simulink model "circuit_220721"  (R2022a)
settings: Solver=VariableStepAuto  StartTime=-D+0.1e-6  StopTime=34e-6  FixedStep=1e-3  MaxStep=0.1e-6  RelTol=1e-3
model workspace (MATLAB code in the model file):
  sGeo = CreateGeometry()
  sConst = CreateConstants()
libraries: fl_lib x9, nesl_utility x3, ee_lib x1

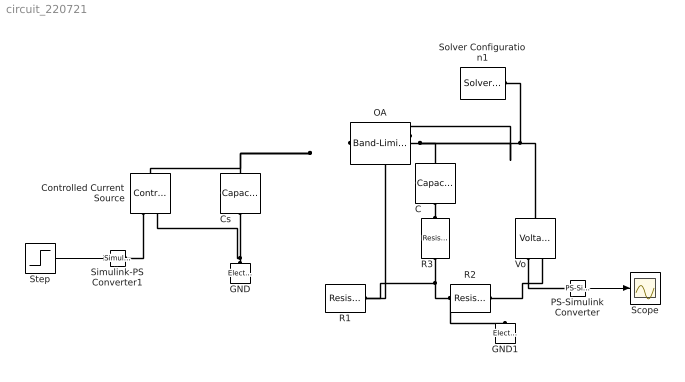
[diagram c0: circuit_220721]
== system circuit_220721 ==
  C : fl_lib/Electrical/Electrical Elements/Capacitor  c=100 uF  r=1e-6 Ohm  g=0 1/Ohm  i_specify=off  i_priority=None  i=0 A  i_nominal_specify=off  i_nominal_unit=A  i_nominal_value=1  v_specify=off  v_priority=None  v=0 V  v_nominal_specify=off  v_nominal_unit=V  v_nominal_value=1  vc_specify=off  vc_priority=High  vc=0 V  vc_nominal_specify=off  vc_nominal_unit=V  vc_nominal_value=1
  Controlled Current Source : fl_lib/Electrical/Electrical Sources/Controlled Current Source
  Cs : fl_lib/Electrical/Electrical Elements/Capacitor  c=33 pF  r=1e-6 Ohm  g=0 1/Ohm  i_specify=off  i_priority=None  i=0 A  i_nominal_specify=off  i_nominal_unit=A  i_nominal_value=1  v_specify=off  v_priority=None  v=0 V  v_nominal_specify=off  v_nominal_unit=V  v_nominal_value=1  vc_specify=off  vc_priority=High  vc=0 V  vc_nominal_specify=off  vc_nominal_unit=V  vc_nominal_value=1
  GND : fl_lib/Electrical/Electrical Elements/Electrical Reference
  GND1 : fl_lib/Electrical/Electrical Elements/Electrical Reference
  OA : ee_lib/Integrated Circuits/Band-Limited Op-Amp  A=100000  Rin=1e8 Ohm  Rout=0 Ohm  Vmin=-15 V  Vmax=15 V  Vdotmax=1000000 V/s  f=1 Hz  V0=0 V
  PS-Simulink Converter : nesl_utility/PS-Simulink Converter  PhysicalDomain=network_engine_domain  SubClassName=ps_output  LeftPortType=input  RightPortType=output  PseudoPeriodic=off  Frequencies=[]  VectorFormat=1-D array  Unit=inherit  AffineConversion=off
  R1 : fl_lib/Electrical/Electrical Elements/Resistor  R=10 MOhm  i_specify=off  i_priority=None  i=0 A  i_nominal_specify=off  i_nominal_unit=A  i_nominal_value=1  v_specify=off  v_priority=None  v=0 V  v_nominal_specify=off  v_nominal_unit=V  v_nominal_value=1
  R2 : fl_lib/Electrical/Electrical Elements/Resistor  R=100 kOhm  i_specify=off  i_priority=None  i=0 A  i_nominal_specify=off  i_nominal_unit=A  i_nominal_value=1  v_specify=off  v_priority=None  v=0 V  v_nominal_specify=off  v_nominal_unit=V  v_nominal_value=1
  R3 : fl_lib/Electrical/Electrical Elements/Resistor  R=1 kOhm  i_specify=off  i_priority=None  i=0 A  i_nominal_specify=off  i_nominal_unit=A  i_nominal_value=1  v_specify=off  v_priority=None  v=0 V  v_nominal_specify=off  v_nominal_unit=V  v_nominal_value=1
  Scope : Scope
  Simulink-PS Converter1 : nesl_utility/Simulink-PS Converter  PhysicalDomain=network_engine_domain  SubClassName=ps_input  LeftPortType=input  RightPortType=output  PseudoPeriodic=off  Frequencies=[]  NoiseDistribution=none  NoiseParameters=[]  Unit=1  AffineConversion=off  FilteringAndDerivatives=provide  SimscapeFilterOrder=1  InputFilterTimeConstant=0.001  UdotUserProvided=0
  Solver Configuration1 : nesl_utility/Solver Configuration  PhysicalDomain=network_engine_domain  SubClassName=solver  LeftPortType=input  RightPortType=generic  Tones=[]  Harmonics=[]  SimulateNoise=off  Profile=off  UseLocalSampling=off  EnableSwitchedLinearOptims=on  FrequencyDomain=off  UseCCode=off  RelTol=0.001  AbsTol=1e-06  MinStep=1e-09  ToWorkspace=off  RevertToSquareIcSolve=off  NumHomotopyIterations=100  PhasorMode=off  PhasorModeNumHarmonics=1  IndexReductionMethod=DerivativeReplacement  DoDC=off  ResidualTolerance=1e-09  UseLocalSolver=off  LocalSolverChoice=NE_BACKWARD_EULER_ADVANCER  LocalSolverSampleTime=0.001  DoFixedCost=off  MaxNonlinIter=3  MaxModeIter=2  ComputeImpulses=off  ImpulseIterations=2  LinearAlgebra=Sparse  LinearAlgebraNumThread=0  EquationFormulation=NE_TIME_EF  DelaysMemoryBudget=1024  AutomaticFiltering=on  FilteringTimeConstant=0.001  PartitionStorageMethod=AS_NEEDED  PartitionMemoryBudget=1024  PartitionMethod=FAST
  Step : Step  SampleTime=0
  Vo : fl_lib/Electrical/Electrical Sensors/Voltage Sensor
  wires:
  Step/1 -> Simulink-PS Converter1/1
  PS-Simulink Converter/1 -> Scope/1
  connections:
  Vo/RConn1 -- PS-Simulink Converter/LConn1
  Solver Configuration1/RConn1 -- Vo/LConn1 -- OA/RConn1 -- OA/LConn2 -- C/LConn1
  Controlled Current Source/RConn1 -- Simulink-PS Converter1/RConn1
  R3/RConn1 -- R1/LConn1 -- R2/RConn1
  R2/LConn1 -- GND1/LConn1 -- Vo/RConn2
  OA/LConn1 -- Cs/LConn1 -- Controlled Current Source/LConn1 -- R1/RConn1
  R3/LConn1 -- C/RConn1
  GND/LConn1 -- Controlled Current Source/RConn2 -- Cs/RConn1
